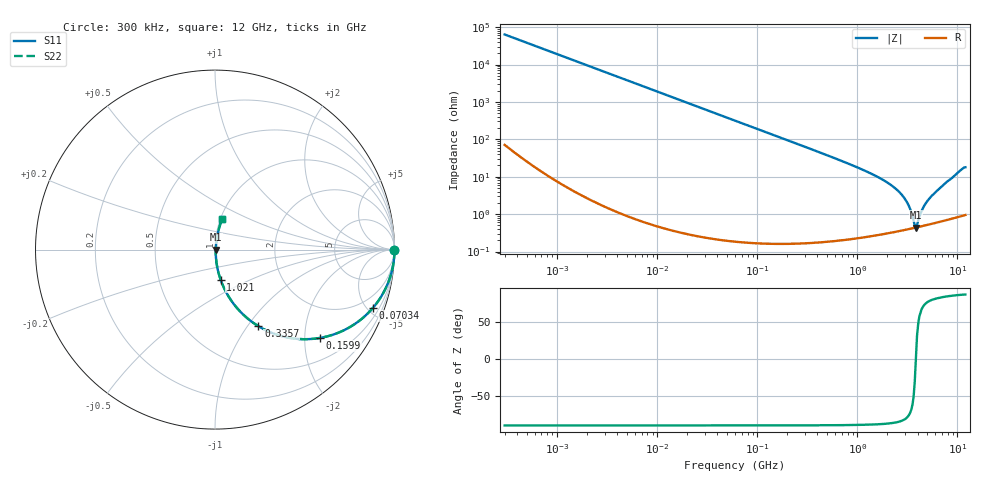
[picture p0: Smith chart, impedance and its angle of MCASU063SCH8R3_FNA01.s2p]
! MCASU063SCH8R3_FNA01  S-PARAMETER MODEL  ( General Type )
! Model Generated by TAIYO YUDEN Corporation (http://www.ty-top.com)
! Version 1.0
! TAIYO YUDEN Control No. 130801
! Copyright(c) 2013 TAIYO YUDEN CO.,LTD. All Rights Reserved.
! Product Description (link to TY-COMPAS)
! https://ds.yuden.co.jp/TYCOMPAS/or/detail?pn=MCASU063SCH8R3DFNA01&u=M
! Products Name : Multilayer Ceramic Capacitors
! Characteristics :
!  Capacitance : 8.3 pF , Rated Voltage : 50V , TCC : CH / C0H
!  Case Size : 0.6 x 0.3 / 0.024 x 0.012 [mm/inch] , Thickness : 0.3 / 0.012 [mm/inch]
!  (Conditions: Temperature = 25 degC , DC Bias Current/Voltage = 0A / 0V)
! External Node Assignments :
!  1  o---| |---o  2
! GND o---------o GND
! Frequency Range : 0.3MHz  -  12000MHz  [ 401 STEP ]
# MHz S RI R 50
! Freq[MHz].  S11 Real  S11 Imag  S21 Real  S21 Imag  S12 Real  S12 Imag  S22 Real  S22 Imag
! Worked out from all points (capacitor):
!   401 points, 300 kHz to 12 GHz, reference 50 ohm
!   read as one part in series: C = 8.35 pF near 316.3 kHz
!   lowest |Z| = 438 mohm at 3.841 GHz (marker M1)
!   series resonance near 3.84 GHz, so ESL is about 210 pH
!   S11 on the Smith chart (normalised r, x): 300 kHz: open; 70.34 MHz: 1.00, -5.42; 159.9 MHz: 1.00, -2.38; 335.7 MHz: 1.00, -1.13; 1.021 GHz: 1.00, -0.35; 12 GHz: 1.02, +0.36
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0.3  1 -0.00157  4.24e-06 0.00157  4.24e-06 0.00157  1 -0.00157
1.769972  0.9999 -0.00928  8.89e-05 0.00928  8.89e-05 0.00928  0.9999 -0.00928
10.44266  0.997 -0.0546  0.003 0.0546  0.003 0.0546  0.997 -0.0546
27.10171  0.9801 -0.1393  0.0199 0.1393  0.0199 0.1393  0.9801 -0.1393
60  0.9097 -0.2863  0.0903 0.2863  0.0903 0.2863  0.9097 -0.2863
70.33673  0.88 -0.3247  0.12 0.3247  0.12 0.3247  0.88 -0.3247
159.8975  0.5861 -0.4919  0.4139 0.4919  0.4139 0.4919  0.5861 -0.4919
335.7268  0.2417 -0.4266  0.7583 0.4266  0.7583 0.4266  0.2417 -0.4266
353.9943  0.2226 -0.4144  0.7774 0.4144  0.7774 0.4144  0.2226 -0.4144
570.2811  0.098 -0.2944  0.902 0.2944  0.902 0.2944  0.098 -0.2944
1021.415  0.0313 -0.1677  0.9687 0.1677  0.9687 0.1677  0.0313 -0.1677
2088.533  0.0072 -0.0637  0.9928 0.0637  0.9928 0.0637  0.0072 -0.0637
2581.562  0.00511 -0.0402  0.9949 0.0402  0.9949 0.0402  0.00511 -0.0402
3026.31  0.00437 -0.0238  0.9956 0.0238  0.9956 0.0238  0.00437 -0.0238
3364.605  0.00421 -0.0132  0.9958 0.0132  0.9958 0.0132  0.00421 -0.0132
3642.919  0.00425 -0.00531  0.9957 0.00531  0.9957 0.00531  0.00425 -0.00531
3841.137  0.00436 2.05e-05  0.9956 -2.05e-05  0.9956 -2.05e-05  0.00436 2.05e-05
4050.141  0.00453 0.00479  0.9955 -0.00479  0.9955 -0.00479  0.00453 0.00479
4623.766  0.00512 0.0153  0.9949 -0.0153  0.9949 -0.0153  0.00512 0.0153
5278.635  0.00599 0.0259  0.994 -0.0259  0.994 -0.0259  0.00599 0.0259
7648.807  0.0114 0.0675  0.9886 -0.0675  0.9886 -0.0675  0.0114 0.0675
12000  0.0396 0.1703  0.9604 -0.1703  0.9604 -0.1703  0.0396 0.1703
